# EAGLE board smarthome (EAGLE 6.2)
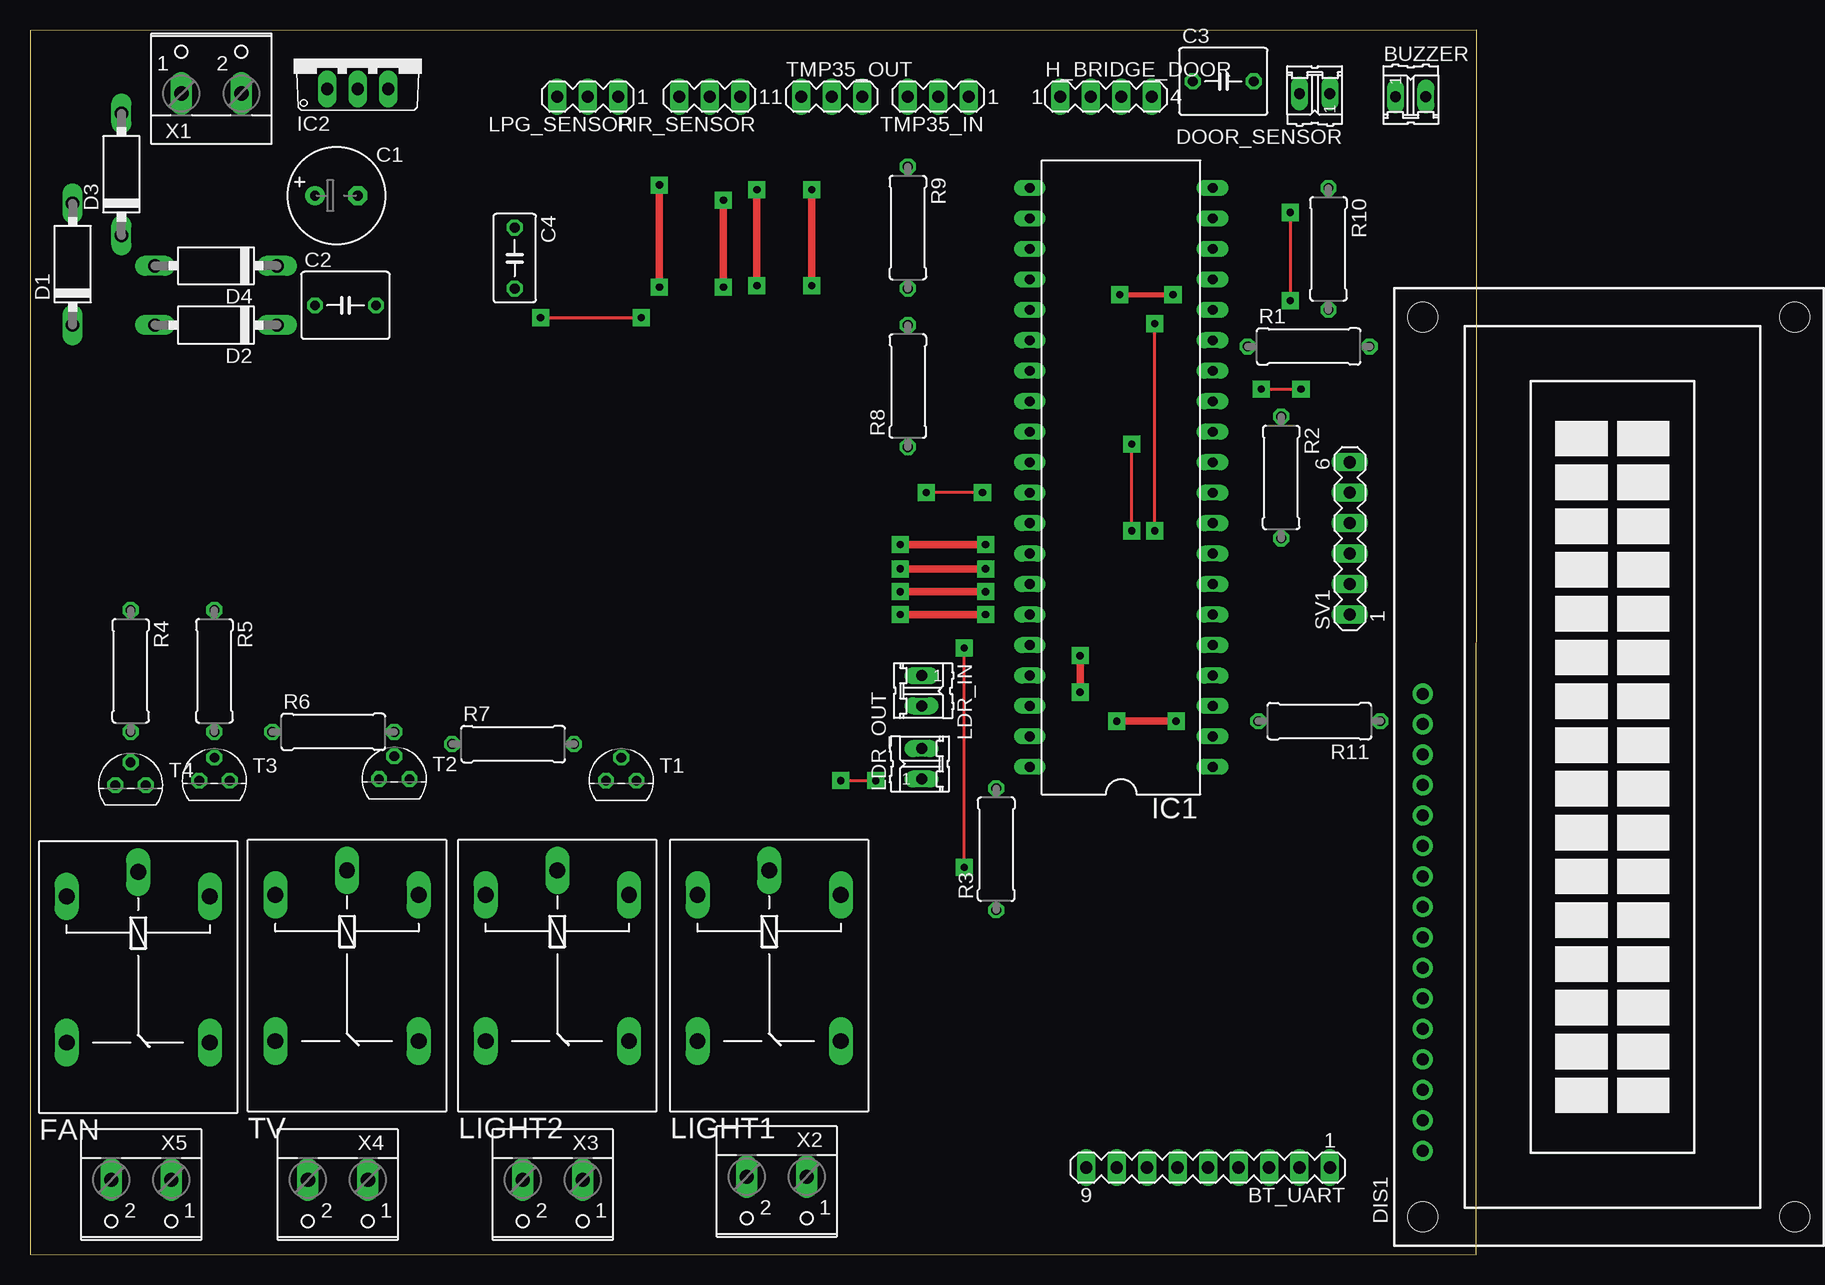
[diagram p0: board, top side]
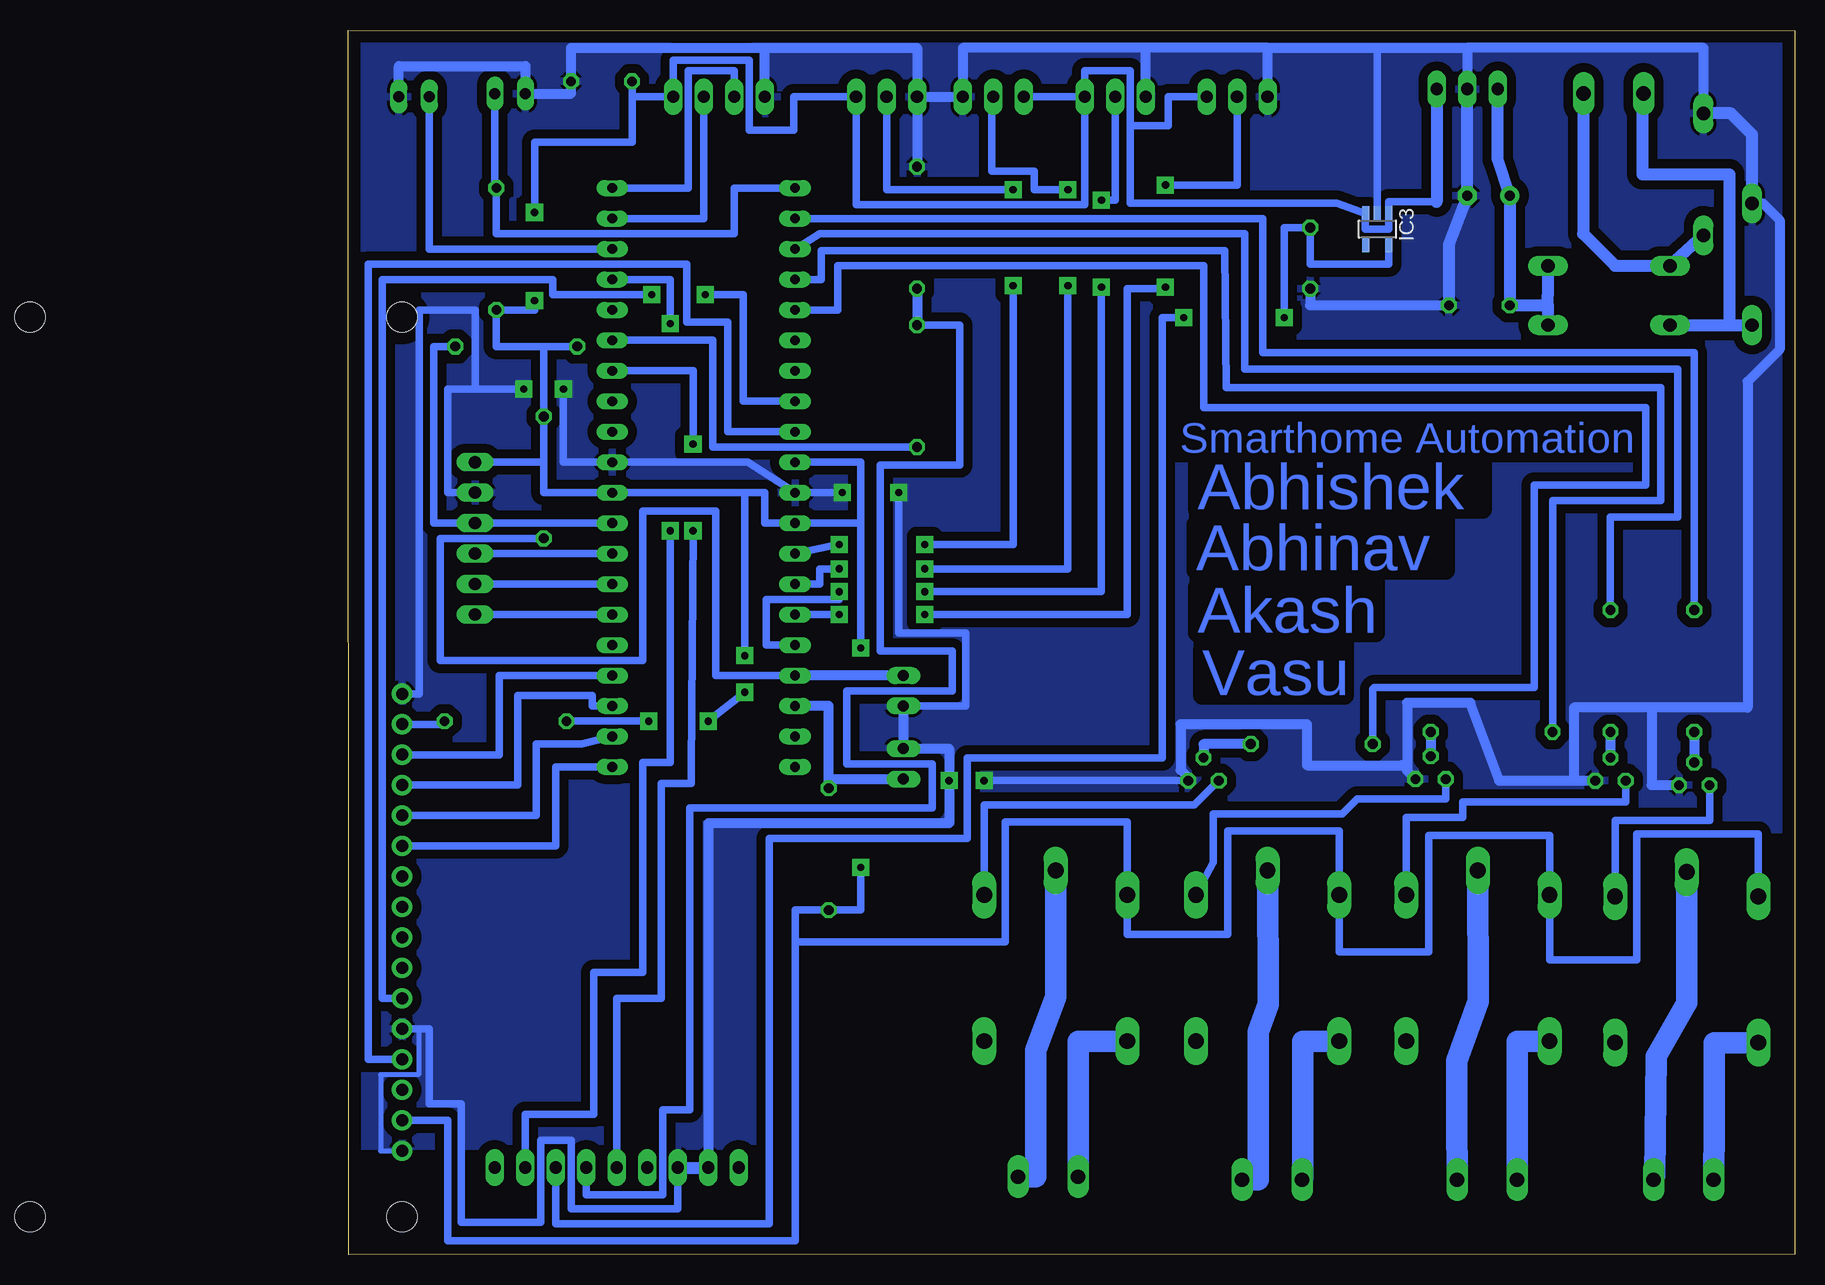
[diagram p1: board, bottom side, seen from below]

Size 120.56 x 102.1 mm. Coordinates in mm from the lower left corner, seen from the top.
Outline: 0,0.03 120.52,0 120.55,102.1 0,102.06 0,0.03
Copper layers (1*16): Top 0.035mm / dielectric 1.5mm / Bottom 0.035mm
Design rules: minimum track width 10mil, minimum drill 24mil, track to track 30mil, track to pad 30mil, pad to pad 8mil, via to via 8mil, smd to smd 8mil, copper to edge 40mil, drill to drill 8mil, minimum pad ring 10mil, minimum via ring 8mil, stop-mask expansion 4mil, vias tented up to drill 0mil, thermal gap 10mil

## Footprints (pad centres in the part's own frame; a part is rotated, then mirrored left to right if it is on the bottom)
MA09-1 = drill 1.016 long: 1 -10.16,0; 2 -7.62,0; 3 -5.08,0; 4 -2.54,0; 5 0,0; 6 2.54,0; 7 5.08,0; 8 7.62,0; 9 10.16,0
02P = drill 0.914 long: 1 -1.27,0; 2 1.27,0
E3,5-8 = drill 0.813 pad 1.6: + -1.778,0 | drill 0.813 pad 1.6 octagon: - 1.778,0
C050-055X075 = drill 0.813 octagon: 1 -2.54,0; 2 2.54,0
C050-035X075 = drill 0.813 octagon: 1 -2.54,0; 2 2.54,0
P1-10 = drill 1.118 long: A 5.08,0; C -5.08,0
TUXGR_16X2_R2 = drill 1 pad 1.676: 1 -32,15.5; 2 -29.46,15.5; 3 -26.92,15.5; 4 -24.38,15.5; 5 -21.84,15.5; 6 -19.3,15.5; 7 -16.76,15.5; 8 -14.22,15.5; 9 -11.68,15.5; 10 -9.14,15.5; 11 -6.6,15.5; 12 -4.06,15.5; 13 -1.52,15.5; 14 1.02,15.5; 15 3.56,15.5; 16 6.1,15.5 | hole 2.5: -37.5,-15.5; 37.5,-15.5; -37.5,15.5; 37.5,15.5
G5LE = drill 1.321 long: 1 -7.493,-5.969; 2 -7.493,5.969; O 4.699,5.969; P -9.525,0; S 4.699,-5.969
MA04-1 = drill 1.016 long: 1 -3.81,0; 2 -1.27,0; 3 1.27,0; 4 3.81,0
DIL40 = drill 0.813 long: 1 -24.13,-7.62; 2 -21.59,-7.62; 3 -19.05,-7.62; 4 -16.51,-7.62; 5 -13.97,-7.62; 6 -11.43,-7.62; 7 -8.89,-7.62; 8 -6.35,-7.62; 9 -3.81,-7.62; 10 -1.27,-7.62; 11 1.27,-7.62; 12 3.81,-7.62; 13 6.35,-7.62; 14 8.89,-7.62; 15 11.43,-7.62; 16 13.97,-7.62; 17 16.51,-7.62; 18 19.05,-7.62; 19 21.59,-7.62; 20 24.13,-7.62; 21 24.13,7.62; 22 21.59,7.62; 23 19.05,7.62; 24 16.51,7.62; 25 13.97,7.62; 26 11.43,7.62; 27 8.89,7.62; 28 6.35,7.62; 29 3.81,7.62; 30 1.27,7.62; 31 -1.27,7.62; 32 -3.81,7.62; 33 -6.35,7.62; 34 -8.89,7.62; 35 -11.43,7.62; 36 -13.97,7.62; 37 -16.51,7.62; 38 -19.05,7.62; 39 -21.59,7.62; 40 -24.13,7.62
TO220V = drill 1.016 long: 1 -2.54,-2.54; 2 0,-2.54; 3 2.54,-2.54
SOT23-5 = smd 0.6 x 1.2: 1 -0.95,-1.306; 2 0,-1.306; 3 0.95,-1.306; 4 0.95,1.306; 5 -0.95,1.306
MA03-1 = drill 1.016 long: 1 -2.54,0; 2 0,0; 3 2.54,0
0309/10 = drill 0.813 octagon: 1 -5.08,0; 2 5.08,0
MA06-1 = drill 1.016 long: 1 -6.35,0; 2 -3.81,0; 3 -1.27,0; 4 1.27,0; 5 3.81,0; 6 6.35,0
TO92 = drill 0.813 octagon: 1 1.27,0; 2 0,1.905; 3 -1.27,0
W237-102 = drill 1.194 long: 1 -2.5,-1.27; 2 2.5,-1.27

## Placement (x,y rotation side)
BT_UART  [MA09-1]  98.17,7.26 180 top
BUZZER  [02P]  115.06,96.55 0 top
C1  1000uF  [E3,5-8]  25.53,88.29 0 top
C2  100nF  [C050-055X075]  26.29,79.15 0 top
C3  100nF  [C050-055X075]  99.44,97.82 0 top
C4  1uf  [C050-035X075]  40.39,83.08 270 top
D1  1N4007  [P1-10]  3.56,82.58 90 top
D2  1N4007  [P1-10]  15.49,77.5 180 top
D3  BA157  [P1-10]  7.62,90.07 90 top
D4  1N4007  [P1-10]  15.49,82.45 180 top
DIS1  TUXGR_16X2_R2  [TUXGR_16X2_R2]  131.57,40.67 90 top
DOOR_SENSOR  [02P]  107.06,96.8 180 top
FAN  G5L  [G5LE]  9.02,22.38 270 top
H_BRIDGE_DOOR  [MA04-1]  89.66,96.55 0 top
IC1  MEGA16-P  [DIL40]  90.93,64.8 90 top
IC2  7805TV  [TO220V]  27.31,99.72 0 top
IC3  LM321MF  [SOT23-5]  34.8,85.5 180 bottom
LDR_IN  [02P]  74.3,47.02 270 top
LDR_OUT  [02P]  74.3,40.92 90 top
LIGHT1  G5L  [G5LE]  61.59,22.5 270 top
LIGHT2  G5L  [G5LE]  43.94,22.5 270 top
LPG_SENSOR  [MA03-1]  46.48,96.55 180 top
PIR_SENSOR  [MA03-1]  56.64,96.55 180 top
R1  [0309/10]  106.55,75.72 0 top
R2  100k  [0309/10]  104.27,64.8 270 top
R3  100k  [0309/10]  80.52,33.81 90 top
R4  4.7k  [0309/10]  8.38,48.67 270 top
R5  4.7k  [0309/10]  15.37,48.67 270 top
R6  4.7k  [0309/10]  25.27,43.59 0 top
R7  4.7k  [0309/10]  40.26,42.57 0 top
R8  5k  [0309/10]  73.15,72.42 90 top
R9  10k  [0309/10]  73.15,85.62 270 top
R10  10k  [0309/10]  108.2,83.85 270 top
R11  220  [0309/10]  107.44,44.48 180 top
SV1  [MA06-1]  109.98,59.72 90 top
T1  BC547  [TO92]  49.28,39.52 0 top
T2  BC547  [TO92]  30.35,39.65 0 top
T3  BC547  [TO92]  15.37,39.52 0 top
T4  BC547  [TO92]  8.38,39.14 0 top
TMP35_IN  [MA03-1]  75.69,96.55 180 top
TMP35_OUT  [MA03-1]  66.8,96.55 0 top
TV  G5L  [G5LE]  26.42,22.5 270 top
X1  9V AC  [W237-102]  15.11,98.07 0 top
X2  [W237-102]  62.23,5.23 180 top
X3  [W237-102]  43.56,4.98 180 top
X4  [W237-102]  25.65,4.98 180 top
X5  [W237-102]  9.27,4.98 180 top

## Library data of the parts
BT_UART H_BRIDGE_DOOR LPG_SENSOR PIR_SENSOR SV1 TMP35_IN TMP35_OUT = con-lstb; OC_FARNELL: unknown; OC_NEWARK: unknown
BUZZER DOOR_SENSOR LDR_IN LDR_OUT = con-amp-quick; OC_FARNELL: unknown; OC_NEWARK: unknown
C1-C4 R1-R11 = resistor
D1-D4 = diode
DIS1 = display-lcd; OC_FARNELL: unknown; OC_NEWARK: unknown
FAN LIGHT1 LIGHT2 TV = relay; OC_FARNELL: unknown; OC_NEWARK: unknown
IC1 = atmel; MPN: ATMEGA16-16PU; OC_FARNELL: 9171142; OC_NEWARK: 01M6885
IC2 IC3 = linear
T1-T4 = transistor
X1-X5 = con-wago-500; MPN: 237-102; OC_FARNELL: unknown; OC_NEWARK: 70K9898

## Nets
+5V: C3.1 DIS1.2 FAN.1 H_BRIDGE_DOOR.4 IC1.10 IC1.30 IC1.32 IC2.3 IC3.1 IC3.3 LIGHT1.1 LIGHT2.1 LPG_SENSOR.1 PIR_SENSOR.1 R1.1 R2.1 R3.1 R10.2 R11.2 SV1.6 TMP35_IN.1 TMP35_OUT.1 TV.1
GND: BT_UART.7 BT_UART.8 BUZZER.2 C1.- C2.2 C3.2 C4.2 D1.A D3.A DIS1.1 DIS1.5 DIS1.16 DOOR_SENSOR.2 H_BRIDGE_DOOR.1 IC1.11 IC1.31 IC2.2 IC3.2 LDR_IN.2 LDR_OUT.2 LPG_SENSOR.3 PIR_SENSOR.3 R9.1 SV1.5 T1.1 T2.1 T3.1 T4.1 TMP35_IN.3 TMP35_OUT.3
N$1: D1.C D2.A X1.1
N$2: D3.C D4.A X1.2
N$3: BT_UART.5 IC1.14
N$4: C1.+ C2.1 D2.C D4.C IC2.1
N$5: BT_UART.4 R8.2 R9.2
N$6: IC1.9 R1.2 SV1.4
N$7: IC1.37 LDR_IN.1 R2.2
N$8: IC1.38 LDR_OUT.1 R3.2
N$9: IC1.33 TMP35_IN.2
N$10: IC1.34 TMP35_OUT.2
N$11: IC1.35 LPG_SENSOR.2
N$12: IC1.36 PIR_SENSOR.2
N$13: IC1.22 R4.1
N$14: IC1.23 R5.1
N$15: IC1.24 R6.1
N$16: IC1.25 R7.1
N$17: R7.2 T1.2
N$18: R6.2 T2.2
N$19: R5.2 T3.2
N$20: R4.2 T4.2
N$21: LIGHT1.2 T1.3
N$22: LIGHT2.2 T2.3
N$23: T3.3 TV.2
N$24: FAN.2 T4.3
N$25: IC1.15 R8.1
N$26: BT_UART.2 IC1.17
N$27: DOOR_SENSOR.1 IC1.21 R10.1
N$28: DIS1.6 IC1.28
N$29: DIS1.4 IC1.29
N$30: DIS1.14 IC1.4
N$31: DIS1.13 IC1.3
N$32: DIS1.12 IC1.2
N$33: DIS1.11 IC1.1
N$34: IC1.6 SV1.1
N$35: BUZZER.1 IC1.18
N$36: IC1.7 SV1.2
N$37: IC1.8 SV1.3
N$38: H_BRIDGE_DOOR.2 IC1.20
N$39: H_BRIDGE_DOOR.3 IC1.19
N$40: LIGHT1.P X2.1
N$41: LIGHT1.S X2.2
N$42: LIGHT2.P X3.1
N$43: LIGHT2.S X3.2
N$44: TV.S X4.2
N$45: TV.P X4.1
N$46: FAN.S X5.2
N$47: FAN.P X5.1
N$48: DIS1.15 R11.1
N$49: BT_UART.3 C4.1 IC3.5

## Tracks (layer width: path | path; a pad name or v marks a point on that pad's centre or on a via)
+5V  (via drill 0.6 pad 1.42)
  Top 0.254: v77.85,32.28 v77.85,50.57 | v105.03,86.89 v105.03,79.53
  Top 0.61: v95.5,44.48 v90.55,44.48 | v87.5,46.89 v87.5,49.94
  Bottom 0.254: DIS1.2
  Bottom 0.61: 87.5,63.53 IC1.10 104.27,63.53 104.27,66.07 | 87.5,63.53 85.85,63.53 85.85,60.99 IC1.32 77.85,60.99 | IC1.30 77.85,66.07 77.85,60.99 | TMP35_OUT.1 PIR_SENSOR.1 | FAN.1 3.05,35.08 13.17,35.08 13.17,24.58 20.45,24.58 TV.1 20.45,34.95 30.52,34.95 30.52,25.25 37.97,25.25 LIGHT2.1 37.97,35.33 47.27,35.33 47.27,26.7 55.63,26.7 LIGHT1.1 55.63,36.09 65.79,36.09 65.79,26.06 83.31,26.06 | 29.84,87.78 33.85,87.78 IC3.1 33.85,85.5 35.81,85.5 35.81,86.8 IC3.3 38.16,87.66 55.37,87.66 55.37,94.13 | LPG_SENSOR.1 52.2,96.55 52.2,94.13 55.37,94.13 | 55.37,94.13 55.37,98.7 59.18,98.7 PIR_SENSOR.1 | 96.9,96.55 H_BRIDGE_DOOR.4 93.47,99.59 87.12,99.59 87.12,93.75 83.44,93.75 83.44,96.55 TMP35_IN.1 78.23,87.53 59.18,87.53 PIR_SENSOR.1 | 96.9,96.55 C3.1 | 83.31,26.06 83.31,1.17 112.27,1.17 112.27,11.2 DIS1.2 | 83.31,26.06 83.31,28.73 R3.1 77.85,28.73 v77.85,32.28 | 104.27,75.72 108.2,75.72 R10.2 105.03,78.77 v105.03,79.53 | 104.27,75.72 R2.1 104.27,66.07 | 104.27,75.72 R1.1 | SV1.6 104.27,66.07 | v77.85,50.57 77.85,60.99 | 96.9,96.55 96.9,92.74 105.03,92.74 v105.03,86.89 | R11.2 v95.5,44.48 | v90.55,44.48 v87.5,46.89 | v87.5,49.94 87.5,63.53
  Bottom 1.016: IC2.3 29.84,87.78
GND  (via drill 0.6 pad 1.42)
  Top 0.254: v67.56,39.52 v70.48,39.52 | v79.38,63.53 v74.68,63.53 | v102.62,72.16 v105.92,72.16
  Bottom 0.254: 114.68,18.83 114.68,18.82 | DIS1.1
  Bottom 0.406: DIS1.5 | 114.68,18.82 114.68,15.01 117.86,15.01 117.86,8.66 DIS1.1
  Bottom 0.61: DIS1.5 114.68,18.83 | 32.77,40.79 32.32,40.35 | BT_UART.7 93.09,3.84 101.98,3.84 101.98,9.55 104.52,9.55 104.52,2.69 111.12,2.69 111.12,12.6 113.79,12.6 113.79,18.82 114.68,18.82 | IC3.2 34.8,100.61 | T1.1 v67.56,39.52 | v79.38,63.53 IC1.31 87.25,66.07 IC1.11 102.62,66.07 v102.62,72.16 | v74.68,63.53 74.68,51.84 69.09,51.84 69.09,45.75 LDR_IN.2 | v105.92,72.16 109.98,72.16 | 109.98,72.16 112.27,72.16 112.27,63.53 SV1.5 | DIS1.16 114.61,46.77 114.61,78.77 109.98,78.77 109.98,72.16
  Bottom 0.813: C4.2 40.39,79.15 C2.2 | BUZZER.2 116.33,99.09 105.79,99.09 DOOR_SENSOR.2 101.98,96.8 C3.2 101.98,100.61 85.85,100.61 | TMP35_IN.3 R9.1 | TMP35_IN.3 TMP35_OUT.3 69.34,100.61 54.1,100.61 | 11.94,45.62 3.94,45.62 3.94,72.8 1.27,75.46 1.27,86.26 2.67,87.66 D1.A | 11.94,45.62 11.94,39.14 T4.1 | 18.41,39.52 18.41,45.62 11.94,45.62 | 18.41,39.52 24.64,39.52 27.05,46 32.32,46 32.32,40.35 T2.1 | 18.41,39.52 T3.1 | 32.77,40.79 40.64,40.79 40.64,44.22 51.18,44.22 51.18,40.41 50.55,39.78 T1.1 | H_BRIDGE_DOOR.1 85.85,100.61 | 85.85,100.61 73.15,100.61 TMP35_IN.3 | 43.94,100.61 34.8,100.61 27.31,100.61 | 27.31,100.61 IC2.2 | LPG_SENSOR.3 43.94,100.61 | 43.94,100.61 54.1,100.61 | PIR_SENSOR.3 54.1,100.61 | LDR_IN.2 LDR_OUT.2 70.48,42.19 v70.48,39.52 70.48,35.97 90.55,35.97 BT_UART.8 | D3.A 7.62,100.61 27.31,100.61
  Bottom 1.016: BT_UART.7 BT_UART.8 | D1.A 3.56,93.37 5.33,95.15 D3.A | IC2.2 C1.- 28.83,84.23 C2.2
  pour Bottom: 0,92.48 -0.13,35.46 67.31,35.33 69.34,32.41 69.34,12.73 69.47,9.04 120.4,9.04 120.52,13.49 120.65,102.39 112.01,102.13 -0.13,102.13
N$1
  Bottom 0.813: X1.1 12.7,96.8
  Bottom 1.016: D2.A 5.46,77.5 | 5.46,77.5 D1.C | 12.7,96.8 12.7,90.07 5.46,90.07 5.46,77.5
N$2
  Bottom 0.813: X1.2 17.65,96.8
  Bottom 1.016: D3.C D4.A 14.99,82.45 17.65,85.12 17.65,96.8
N$3  (via drill 0.6 pad 1.42)
  Top 0.254: v91.82,60.35 v91.82,67.59
  Bottom 0.61: BT_UART.5 98.17,21.36 94.49,21.36 94.49,39.27 91.95,39.27 91.95,40.41 v91.82,60.35 | v91.82,67.59 91.82,73.69 IC1.14
N$4
  Bottom 1.016: D4.C 20.57,80.04 20.57,79.15 | 20.57,79.15 D2.C | 20.57,79.15 C2.1 C1.+ 24.77,91.34 IC2.1
N$5
  Bottom 0.61: BT_UART.4 100.71,4.98 94.36,4.98 94.36,12.09 92.08,12.09 92.08,37.24 71.88,37.24 71.88,40.92 78.99,40.92 78.99,47.02 70.23,47.02 70.23,50.32 76.2,50.32 76.2,65.81 69.6,65.81 69.6,77.5 R8.2
  Bottom 0.813: R9.2 R8.2
N$6
  Bottom 0.61: IC1.9 SV1.4 113.41,60.99 113.41,75.72 R1.2
N$7
  Bottom 0.61: IC1.37 89.92,48.29 89.92,62 96.01,62 96.01,49.56 112.9,49.56 112.9,59.72 R2.2
  Bottom 0.813: LDR_IN.1 IC1.37
N$8
  Bottom 0.813: 80.52,39.65 80.52,45.75 IC1.38 | R3.2 80.52,39.65 | 80.52,39.65 LDR_OUT.1
N$9  (via drill 0.6 pad 1.42)
  Top 0.61: v65.15,88.8 v65.15,80.8 | v72.52,59.21 v79.63,59.21
  Bottom 0.61: TMP35_IN.2 75.69,88.8 v65.15,88.8 | v65.15,80.8 65.15,59.21 v72.52,59.21 | v79.63,59.21 79.76,59.21 IC1.33
N$10  (via drill 0.6 pad 1.42)
  Top 0.61: v60.58,88.8 v60.58,80.8 | v79.63,57.18 v72.52,57.18
  Bottom 0.61: TMP35_OUT.2 66.93,96.55 66.93,90.32 63.37,90.32 63.37,88.8 v60.58,88.8 | IC1.34 81.28,55.91 81.28,57.18 v79.63,57.18 | v72.52,57.18 60.58,57.18 v60.58,80.8
N$11  (via drill 0.6 pad 1.42)
  Top 0.61: v52.45,89.18 v52.45,80.67 | v79.63,53.37 v72.52,53.37
  Bottom 0.61: LPG_SENSOR.2 46.48,92.48 46.48,89.18 v52.45,89.18 | IC1.35 v79.63,53.37 | v72.52,53.37 55.63,53.37 55.63,80.54 52.45,80.54 v52.45,80.67
N$12  (via drill 0.6 pad 1.42)
  Top 0.61: v57.78,87.91 v57.78,80.67 | v79.63,55.27 v72.52,55.27
  Bottom 0.61: PIR_SENSOR.2 56.64,87.91 v57.78,87.91 | IC1.36 85.72,50.83 85.72,54.64 79.63,54.64 v79.63,55.27 | v72.52,55.27 57.78,55.27 v57.78,80.67
N$13
  Bottom 0.61: R4.1 8.38,75.21 44.32,75.21 44.32,86.39 IC1.22
N$14
  Bottom 0.61: R5.1 15.37,61.49 9.78,61.49 9.78,73.81 45.85,73.81 45.85,85.12 81.28,85.12 IC1.23
N$15
  Bottom 0.61: R6.1 20.19,62.89 11.18,62.89 11.18,72.29 47.37,72.29 47.5,83.72 81.15,83.72 81.15,81.31 IC1.24
N$16
  Bottom 0.61: IC1.25 79.76,78.77 79.76,82.45 49.28,82.45 49.28,70.64 12.45,70.64 12.45,64.16 21.72,64.16 21.72,47.27 35.05,47.27 35.18,47.14 R7.1
N$17
  Bottom 0.813: R7.2 49.28,42.57 T1.2
N$18
  Bottom 0.813: R6.2 T2.2
N$19
  Bottom 0.813: R5.2 T3.2
N$20
  Bottom 0.813: R4.2 T4.2
N$21
  Bottom 0.61: T1.3 50.04,37.49 67.56,37.49 LIGHT1.2
N$22
  Bottom 0.61: T2.3 29.08,38 36.45,38 37.72,36.73 48.49,36.76 48.49,32.69 LIGHT2.2
N$23
  Bottom 0.61: T3.3 14.1,37.74 27.69,37.74 27.69,36.47 32.39,36.47 TV.2
N$24
  Bottom 0.61: T4.3 7.11,36.22 14.99,36.22 FAN.2
N$25
  Bottom 0.61: R8.1 90.17,67.34 90.17,76.23 IC1.15
N$26  (via drill 0.6 pad 1.42)
  Top 0.254: v93.73,60.35 v93.73,77.62
  Bottom 0.61: BT_UART.2 105.79,11.71 100.08,11.71 100.08,23.52 96.01,23.52 96.01,41.05 93.73,41.05 v93.73,60.35 | v93.73,77.62 93.73,81.31 IC1.17
N$27
  Bottom 0.254: R10.1 108.33,88.93
  Bottom 0.61: 108.33,88.93 DOOR_SENSOR.1 | R10.1 108.2,85.12 88.39,85.12 88.39,88.93 IC1.21
N$28  (via drill 0.6 pad 1.42)
  Top 0.406: v90.8,80.04 v95.25,80.04
  Bottom 0.61: IC1.28 87.63,71.15 87.63,80.04 v90.8,80.04 | v95.25,80.04 103.51,80.04 103.51,81.31 117.73,81.31 117.73,21.36 DIS1.6
N$29
  Bottom 0.61: IC1.29 88.92,68.61 88.92,77.75 92.33,77.75 92.33,82.58 118.87,82.58 118.87,16.28 116.33,16.28 DIS1.4
N$30
  Bottom 0.254: DIS1.14
  Bottom 0.61: IC1.4 107.95,48.29 107.95,41.68 DIS1.14
N$31
  Bottom 0.254: DIS1.13
  Bottom 0.61: IC1.3 100.2,45.75 100.2,46.63 106.43,46.63 106.43,39.14 DIS1.13
N$32
  Bottom 0.254: DIS1.12
  Bottom 0.61: IC1.2 101.09,42.57 104.9,42.57 104.9,36.6 DIS1.12
N$33
  Bottom 0.254: DIS1.11
  Bottom 0.61: IC1.1 103.25,40.67 103.25,34.06 DIS1.11
N$34
  Bottom 0.61: SV1.1 IC1.6
N$35
  Bottom 0.61: IC1.18 113.79,83.85 BUZZER.1
N$36
  Bottom 0.61: SV1.2 IC1.7
N$37
  Bottom 0.61: SV1.3 IC1.8
N$38
  Bottom 0.61: H_BRIDGE_DOOR.2 88.39,98.7 92.2,98.7 92.2,88.93 IC1.20
N$39
  Bottom 0.61: IC1.19 90.93,86.39 H_BRIDGE_DOOR.3
N$40
  Bottom 1.778: X2.1 63.25,6.5 63.25,17.04 61.59,21.49 LIGHT1.P
N$41
  Bottom 1.778: LIGHT1.S 59.73,17.81 X2.2
N$42
  Bottom 1.778: LIGHT2.P 43.9,20.85 44.7,18.57 44.7,6.25 X3.1
N$43
  Bottom 1.778: X3.2 41.02,6.38 41.02,17.81 LIGHT2.S
N$44
  Bottom 0.406: X4.2 23.11,6.25
  Bottom 1.778: 23.11,6.25 23.11,17.81 TV.S
N$45
  Bottom 1.778: TV.P 26.38,21.11 28.19,16.15 28.19,11.2 X4.1
N$46
  Bottom 1.778: X5.2 6.73,10.82 6.73,17.68 FAN.S
N$47
  Bottom 1.27: X5.1 11.68,6.63
  Bottom 1.778: 11.68,6.63 11.56,16.54 9.02,20.98 FAN.P
N$48
  Bottom 0.61: R11.1 112.65,44.48 112.65,44.22 DIS1.15
N$49  (via drill 0.6 pad 1.42)
  Top 0.254: v42.55,78.13 v50.93,78.13
  Bottom 0.61: IC3.5 33.84,83.3 33.84,82.58 40.39,82.58 C4.1 42.55,85.62 v42.55,78.13 | v50.93,78.13 52.7,78.13 52.7,41.43 68.96,41.43 68.96,34.7 85.47,34.7 85.47,2.57 103.25,2.57 BT_UART.3

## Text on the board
Bottom: Smarthome Automation | Abhishek | Abhinav | Akash | Vasu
